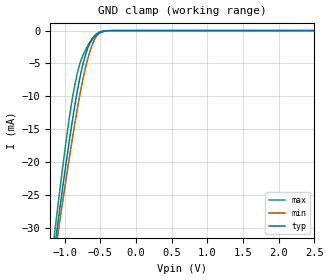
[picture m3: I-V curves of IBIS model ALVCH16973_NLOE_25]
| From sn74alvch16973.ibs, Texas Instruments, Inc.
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[Model]   ALVCH16973_NLOE_25
Model_type  Input
Vinl=0.7
Vinh=1.7
| variable   typ   min   max
C_comp   2.42pF   2.00pF   2.99pF
[Temperature Range]   40   100   -40
| Ambient temperature   25   85   -40
[Voltage range]   2.5   2.3   2.7
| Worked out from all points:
|   GND clamp passes 1 mA (typ) near -0.58 V on its own axis
[GND Clamp]
| ALVCH16973_NLOE_25
|   Voltage   I(typ)   I(min)   I(max)
-2.5V     -154.3mA   -145.9mA   -164.5mA
-1.145V   -33.47mA   -34.86mA   -31.33mA
-1.105V   -30.2mA    -31.85mA   -27.72mA
-1.085V   -28.58mA   -30.35mA   -25.93mA
-930mV    -16.54mA   -19.13mA   -13.04mA
-820mV    -9.124mA   -11.84mA   -6.44mA
-745mV    -5.25mA    -7.527mA   -3.847mA
-675mV    -2.681mA   -4.31mA    -2.304mA
-595mV    -1.134mA   -1.719mA   -967.5uA
-525mV    -460.2uA   -548.5uA   -284.1uA
-340mV    -6.934uA   -11.01uA   -976nA
2.5V      156.4pA    884.6pA    34.32pA
